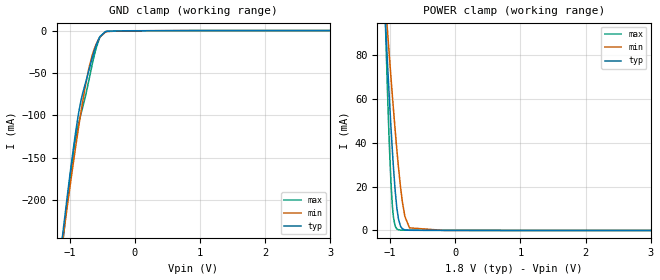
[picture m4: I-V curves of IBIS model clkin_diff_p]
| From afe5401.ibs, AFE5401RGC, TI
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|   clkin_diff Model
[Model]   clkin_diff_p
Model_type   Input
Vinl = 0.45
Vinh = 1.35
|   (nom PVT)   (fast PVT)   (slow PVT)
C_comp   2.874e-12   2.445e-12   3.305e-12
[Model spec]
|subparameter
Vinl   0.45   0.425   0.475
Vinh   1.35   1.275   1.425
| Where nom  PVT is Nominal Process, 1.8V, 27C
|   Fast PVT is Strong Process,  1.9V, -40C
|   Slow PVT is Weak Process,   1.7V, 125C
[Voltage Range]   1.8   1.7   1.9
|Junction Temperature
[Temperature Range]   27   125   -40
[Power Clamp Reference]   1.8   1.7   1.9
[GND Clamp Reference]   0   0   0
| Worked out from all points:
|   GND clamp passes 1 mA (typ) near -0.43 V on its own axis
|   POWER clamp passes 1 mA (typ) near -0.82 V on its own axis
[GND Clamp]
|   Voltage   I(typ)   I(min)   I(max)
-1.8V     -724.5mA   -669.9mA   -781.7mA
-1.125V   -253mA     -258.8mA   -264.9mA
-1.029V   -191mA     -203.5mA   -197.5mA
-967.8mV  -154.2mA   -170mA     -158.8mA
-920.3mV  -127.1mA   -144.4mA   -132.9mA
-870.1mV  -101.4mA   -118.4mA   -112.5mA
-820.8mV  -81.09mA   -93.99mA   -96.95mA
-749.3mV  -60.24mA   -61.93mA   -75.16mA
-647.4mV  -30.98mA   -27.95mA   -38.26mA
-544.1mV  -8.568mA   -8.924mA   -9.663mA
-449.1mV  -1.316mA   -1.856mA   -1.251mA
3.6V      0A         0A         0A
[POWER Clamp]
|   Voltage   I(typ)   I(min)   I(max)
-1.8V     579.6mA    427.8mA    962.7mA
-1.074V   95.6mA     104.3mA    95.01mA
-1.042V   76.6mA     91.04mA    63.8mA
-1.008V   57.5mA     77.38mA    35.23mA
-986.8mV  46.46mA    69.2mA     21.3mA
-948.6mV  28.26mA    54.73mA    5.854mA
-895.6mV  9.817mA    36.11mA    658.9uA
-873mV    5.272mA    28.91mA    307.4uA
-813.6mV  787.6uA    13.21mA    129.6uA
-774.9mV  260uA      6.451mA    117.4uA
-703.5mV  93.83uA    1.193mA    109.4uA
3.6V      0A         0A         0A
